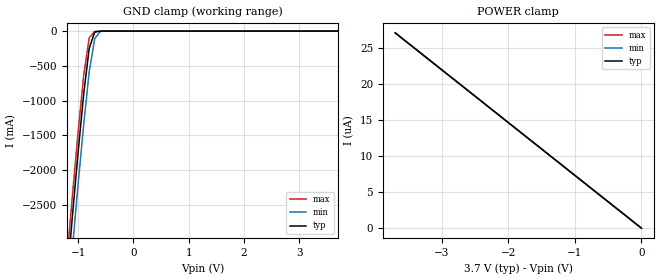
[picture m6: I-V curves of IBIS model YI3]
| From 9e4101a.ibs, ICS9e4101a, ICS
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|   Model YI3
[Model]   YI3
Model_type   Input
Polarity   Non-Inverting
Enable   Active-High
Vinl =   0.80V
Vinh =   2.00V
C_comp   5.50pF   5.00pF   6.00pF
[Temperature Range]   27.00   70.00   0.000
[Voltage Range]   3.70V   3.00V   3.70V
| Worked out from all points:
|   GND clamp passes 1 mA (typ) near -0.60 V on its own axis
[GND_clamp]
| voltage   I(typ)   I(min)   I(max)
-3.7V     -28.01A    -28.44A    -27.75A
-1.2V     -3.55A     -4.02A     -3.26A
-1.1V     -2.63A     -3.1A      -2.34A
-1V       -1.74A     -2.2A      -1.45A
-900mV    -910mA     -1.35A     -640mA
-800mV    -250mA     -590mA     -96.86mA
-700mV    -14.61mA   -110mA     -3.9mA
-600mV    -910uA     -5.85mA    -480uA
-500mV    -120uA     -380uA     -75.89uA
3.7V      140pA      5.13uA     130pA
[POWER_clamp]
| voltage   I(typ)   I(min)   I(max)
-3.7V     27.13uA    27.13uA    27.13uA
-3V       21.99uA    22uA       21.99uA
-2.7V     19.8uA     19.8uA     19.8uA
0V        140pA      310pA      130pA
